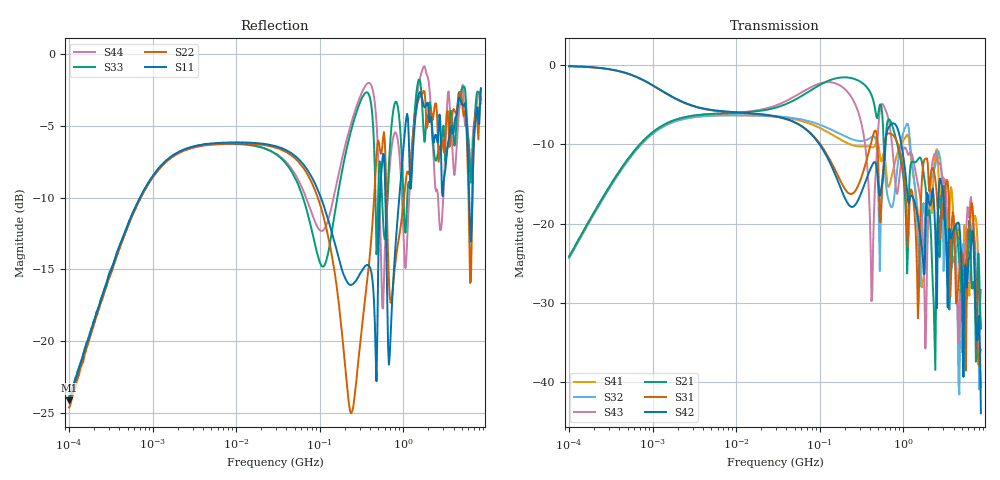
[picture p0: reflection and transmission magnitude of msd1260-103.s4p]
# MHz S MA R 50
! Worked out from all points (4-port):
!   498 points, 100 kHz to 8.5 GHz, reference 50 ohm
!   strongest paths, dB at 100 kHz, 1.698 MHz, 29.49 MHz, 500.7 MHz, 8.5 GHz:
!     S42: -0.1, -3.9, -6.4, -15.1, -44.0
!     S31: -0.1, -4.0, -6.5, -11.9, -40.7
!     S21: -24.2, -7.0, -5.4, -6.2, -33.3
!     S43: -24.2, -7.1, -5.1, -8.2, -28.4
!     S32: -24.3, -7.2, -6.4, -14.8, -35.9
!     S41: -24.3, -7.2, -6.5, -9.9, -33.0
!   lowest |S11| = -24.1 dB at 100 kHz (marker M1), VSWR 1.13, Z = 50.3 + j6.23 ohm
!   |S11| at or under -10 dB: 103.2 MHz to 526.5 MHz (423.3 MHz wide, 134 % of centre); 610.6 MHz to 896 MHz (285.4 MHz wide, 37.9 % of centre); 6.161 GHz to 6.712 GHz (550.9 MHz wide, 8.56 % of centre)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
0.1  0.06209 83.3  0.06201 81.2  0.9866 -3.6  0.06061 -99.2
     0.06201 81.2  0.0586 82.5  0.06061 -99.1  0.988 -3.5
     0.9866 -3.6  0.06061 -99.1  0.06412 83.8  0.06184 81.1
     0.06061 -99.2  0.988 -3.5  0.06184 81.1  0.06213 83.7
7.491482  0.4915 2.3  0.4979 8.3  0.5077 -13.7  0.483 178.4
          0.4979 8.3  0.4876 1.7  0.4832 177.6  0.5114 -13.6
          0.5077 -13.7  0.4832 177.6  0.4884 1.7  0.4981 8.2
          0.483 178.4  0.5114 -13.6  0.4981 8.2  0.4856 2.5
220.0307  0.1586 -43.3  0.8365 -38.1  0.156 166.5  0.32 32.6
          0.8365 -38.1  0.0629 -50.7  0.3483 19.2  0.1325 166.5
          0.156 166.5  0.3483 19.2  0.4957 8.3  0.67 -69.9
          0.32 32.6  0.1325 166.5  0.67 -69.9  0.5297 1.9
1840.304  0.6557 -162.1  0.1741 98.0  0.2563 -169.7  0.06103 -153.4
          0.1741 98.0  0.6876 -169.2  0.06247 159.5  0.0892 -146.1
          0.2563 -169.7  0.06247 159.5  0.5257 -158.3  0.01622 1.0
          0.06103 -153.4  0.0892 -146.1  0.01622 1.0  0.8909 -170.9
3488.216  0.497 21.8  0.03031 -136.3  0.1518 -84.8  0.04197 83.8
          0.03031 -136.3  0.5577 4.1  0.02931 -18.5  0.07609 33.1
          0.1518 -84.8  0.02931 -18.5  0.4929 26.3  0.04683 -89.6
          0.04197 83.8  0.07609 33.1  0.04683 -89.6  0.7417 11.2
5898.28  0.476 -139.4  0.05547 84.5  0.09187 -169.4  0.03886 167.5
         0.05547 84.5  0.4077 -152.4  0.08785 -151.2  0.04438 152.0
         0.09187 -169.4  0.08785 -151.2  0.5245 -144.0  0.1271 84.8
         0.03886 167.5  0.04438 152.0  0.1271 84.8  0.552 -129.4
8500  0.7572 -38.7  0.02165 -119.6  0.009246 155.8  0.02235 -161.8
      0.02165 -119.6  0.7623 -46.2  0.01596 -143.3  0.006315 88.3
      0.009246 155.8  0.01596 -143.3  0.6923 -54.1  0.03811 -23.2
      0.02235 -161.8  0.006315 88.3  0.03811 -23.2  0.6732 -55.3
